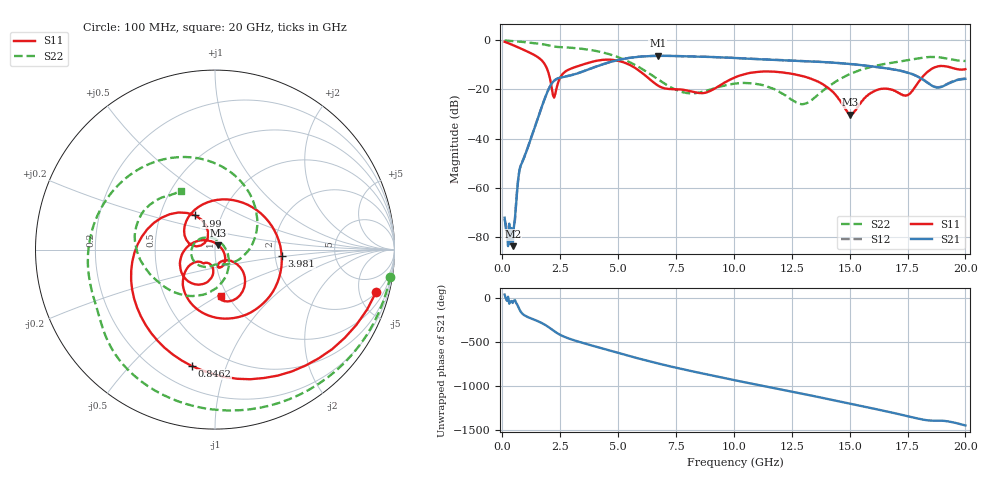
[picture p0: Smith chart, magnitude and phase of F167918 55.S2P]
!  2-Port S-parameters saved by WinCal
! VAR MeasName=S-Parameters (CALIBRATED_DATA) read from VNA (N5242A)
! VAR MeasDate=2016-11-22 10:27:30
! VAR NAME=F167918 55
! VAR FILENAME=F167918 55.S2P
! VAR DATE=2016-11-22 10:27:30
! VAR PHYS_PORTS=1,2
# Hz S DB R 50
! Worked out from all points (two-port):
!   401 points, 100 MHz to 20 GHz, reference 50 ohm
!   highest |S21| = -6.34 dB at 6.717 GHz (marker M1); lowest = -83.8 dB at 448.2 MHz (marker M2)
!   |S21| within 3 dB of the highest: 4.491 GHz to 14.61 GHz (10.12 GHz wide, 106 % of centre)
!   lowest |S11| = -30.3 dB at 15.03 GHz (marker M3), VSWR 1.06, Z = 51.8 + j2.56 ohm
!   |S11| at or under -10 dB: 1.848 GHz to 3.445 GHz (1.598 GHz wide, 60.4 % of centre); 5.493 GHz to end of sweep
!   |S22| runs from -26.1 to -0.1 dB; largest |S21 - S12| = 0.0036
!   S11 on the Smith chart (normalised r, x): 100 MHz: 2.08, -7.12; 846.2 MHz: 0.33, -0.76; 1.99 GHz: 0.75, +0.30; 3.981 GHz: 2.17, -0.19; 20 GHz: 0.93, -0.51
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1e8  -0.65 -14.8  -72.20 33.9  -72.80 50.4  -0.10 -8.8
4.4825e8  -1.91 -57.8  -83.78 -61.6  -78.81 -28.2  -0.33 -37.0
8.4625e8  -3.59 -101.4  -49.96 -177.5  -49.76 -177.0  -0.67 -67.1
1.44325e9  -6.34 -165.7  -34.20 101.5  -34.17 101.5  -1.27 -107.1
1.9905e9  -13.14 120.1  -20.14 25.5  -20.12 25.6  -2.08 -139.0
2.23925e9  -23.36 146.0  -16.50 -21.8  -16.48 -21.7  -2.57 -150.5
2.63725e9  -13.42 142.5  -14.97 -81.3  -14.95 -81.2  -2.87 -167.2
3.43325e9  -10.04 48.3  -12.88 -152.6  -12.87 -152.6  -3.48 157.1
3.9805e9  -8.55 -5.8  -10.97 166.2  -10.96 166.3  -4.25 131.8
5.274e9  -9.11 -105.1  -7.53 70.7  -7.49 70.7  -7.93 67.8
6.71675e9  -18.41 -145.7  -6.34 -28.8  -6.35 -28.8  -15.86 -13.1
6.7665e9  -18.69 -144.8  -6.35 -31.9  -6.35 -32.0  -16.17 -16.3
8.06e9  -20.62 -127.1  -6.56 -110.0  -6.56 -110.1  -21.58 -81.1
9.055e9  -20.29 -99.0  -6.83 -166.2  -6.82 -166.2  -19.88 -110.7
1.005e10  -15.11 -100.8  -7.22 139.3  -7.21 139.4  -17.65 -145.9
1.139325e10  -12.71 -132.6  -7.87 68.5  -7.82 68.4  -18.69 159.0
1.338325e10  -15.89 177.1  -8.63 -36.4  -8.62 -36.6  -24.18 -0.7
1.5025e10  -30.28 53.9  -9.69 -126.1  -9.70 -126.3  -13.69 -84.8
1.67165e10  -19.94 -77.1  -11.58 138.7  -11.63 139.0  -9.34 -139.8
1.75125e10  -22.35 -54.1  -13.20 90.9  -13.15 91.2  -8.14 -161.7
1.875625e10  -10.76 -61.1  -19.23 39.9  -19.09 40.4  -6.84 154.4
2e10  -11.77 -82.7  -15.72 -13.9  -15.59 -13.9  -8.43 120.4
